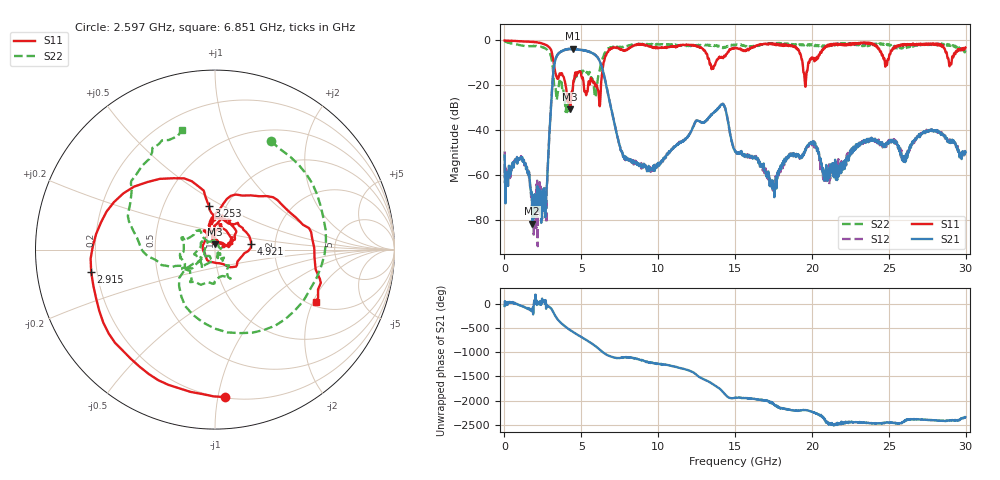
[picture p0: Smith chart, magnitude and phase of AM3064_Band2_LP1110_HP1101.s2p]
# Hz S DB R 50.0
!freq dBS11 angS11 dBS21 angS21 dBS12 angS12 dBS22 angS22
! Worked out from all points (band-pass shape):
!   1600 points, 10 MHz to 29.98 GHz, reference 50 ohm
!   highest |S21| = -3.69 dB at 4.434 GHz (marker M1); lowest = -81.6 dB at 1.809 GHz (marker M2)
!   |S21| within 3 dB of the highest: 3.429 GHz to 5.928 GHz (2.499 GHz wide, 53.4 % of centre); 5.947824 GHz to 5.952211 GHz (4.387 MHz wide, 0.0737 % of centre)
!   lowest |S11| = -30.7 dB at 4.284 GHz (marker M3), VSWR 1.06, Z = 49.8 + j2.92 ohm
!   |S11| at or under -10 dB: 3.206 GHz to 6.444 GHz (3.238 GHz wide, 67.1 % of centre); 13.34 GHz to 13.73 GHz (395.7 MHz wide, 2.92 % of centre); 19.39 GHz to 19.76 GHz (372.2 MHz wide, 1.9 % of centre)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
!   |S22| runs from -32.4 to -0.3 dB; largest |S21 - S12| = 0.019
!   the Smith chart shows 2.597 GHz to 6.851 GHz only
!   S11 on the Smith chart (normalised r, x): 2.597 GHz: 0.21, -1.05; 2.915 GHz: 0.18, -0.09; 3.253 GHz: 0.83, +0.43; 4.921 GHz: 1.50, +0.09; 6.851 GHz: 2.17, -2.11
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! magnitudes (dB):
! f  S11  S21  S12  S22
! 10 MHz  0.0  -51.4  -49.5  -0.3
! 1.191 GHz  -0.4  -54.1  -53.6  -2.3
! 1.809 GHz  -0.6  -81.6  -71.5  -2.5
! 2.597 GHz  -1.7  -74.2  -74.8  -3.4
! 2.915 GHz  -3.1  -42.5  -42.7  -5.2
! 3.253 GHz  -12.2  -10.4  -10.2  -21.1
! 4.284 GHz  -30.7  -3.9  -3.7  -28.7
! 4.434 GHz  -22.3  -3.7  -3.8  -22.5
! 4.921 GHz  -13.8  -4.2  -4.0  -13.2
! 5.015 GHz  -16.0  -4.2  -4.2  -14.4
! 6.139 GHz  -24.4  -8.5  -8.4  -15.1
! 6.851 GHz  -4.0  -27.4  -27.4  -3.2
! 7.826 GHz  -4.7  -52.1  -52.7  -2.9
! 10 GHz  -3.4  -54.5  -55.6  -1.8
! 14.14 GHz  -7.5  -28.4  -28.4  -3.0
! 15 GHz  -3.2  -49.2  -49.5  -1.9
! 17.48 GHz  -1.5  -63.9  -64.0  -1.2
! 19.56 GHz  -20.4  -48.7  -49.0  -1.9
! 19.99 GHz  -7.6  -45.4  -45.8  -1.7
! 20.87 GHz  -2.7  -59.0  -61.2  -2.7
! 25 GHz  -8.3  -45.2  -44.4  -1.7
! 29.98 GHz  -3.2  -49.9  -50.2  -4.5
